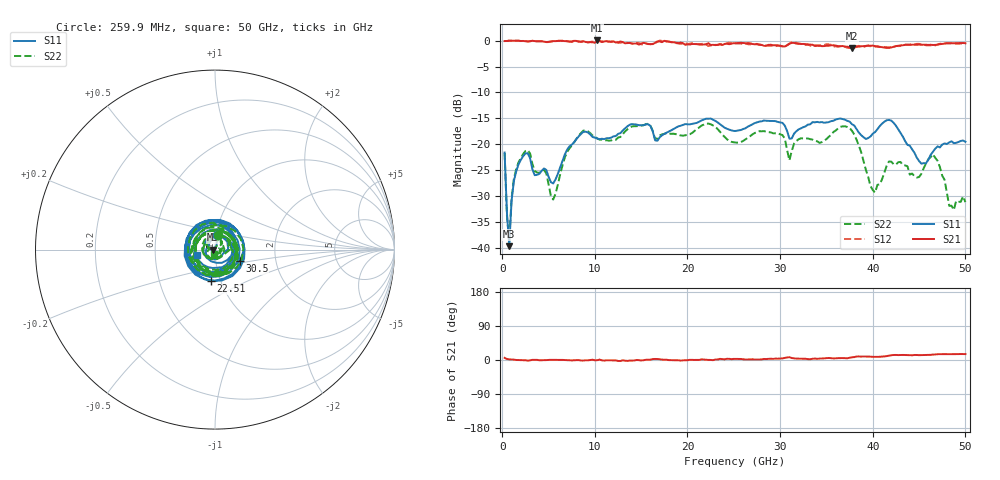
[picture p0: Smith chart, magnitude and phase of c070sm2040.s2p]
! 7/29/2020 12:24:18 PM
! D:\C070SM2040.S2P
! CHANNEL.1
! TR.MEASUREMENT
! CORRECTED.DATA
# GHZ S RI R 50.0
! FREQ.GHZ  S11RE  S11IM  S21RE  S21IM  S12RE  S12IM  S22RE  S22IM
!; PortSelection: Port_12
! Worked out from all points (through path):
!   200 points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, 259.9 MHz to 50 GHz, reference 50 ohm
!   highest |S21| = 0.03 dB at 10.26 GHz (marker M1); lowest = -1.5 dB at 37.75 GHz (marker M2)
!   lowest |S11| = -39.7 dB at 759.9 MHz (marker M3), VSWR 1.02, Z = 49 + j0.0382 ohm
!   |S11| at or under -10 dB: start of sweep to end of sweep
!   |S22| runs from -38.7 to -16.0 dB; largest |S21 - S12| = 0.057
!   S11 on the Smith chart (normalised r, x): 259.9 MHz: 1.01, +0.17; 22.51 GHz: 0.90, -0.33; 30.5 GHz: 1.31, -0.17; 50 GHz: 0.81, -0.05
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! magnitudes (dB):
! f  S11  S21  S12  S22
! 259.9 MHz  -21.6  -0.1  -0.1  -21.7
! 509.9 MHz  -33.2  -0.1  -0.1  -33.7
! 759.9 MHz  -39.7  0.0  0.0  -38.7
! 1.26 GHz  -27.1  0.0  0.0  -26.7
! 2.26 GHz  -22.3  -0.1  -0.1  -21.9
! 4.759 GHz  -25.0  -0.3  -0.3  -25.6
! 5.509 GHz  -27.6  -0.1  -0.1  -30.7
! 8.758 GHz  -17.6  -0.1  -0.2  -17.4
! 10.26 GHz  -18.9  0.0  -0.3  -18.9
! 17.01 GHz  -18.7  -0.2  0.0  -18.3
! 22.51 GHz  -15.0  -0.9  -0.9  -16.1
! 25.25 GHz  -17.4  -0.5  -0.5  -19.7
! 30.5 GHz  -16.4  -1.1  -1.1  -18.9
! 31 GHz  -18.9  -0.6  -0.6  -23.1
! 33.5 GHz  -15.7  -0.8  -1.0  -19.1
! 37.75 GHz  -16.1  -1.5  -1.2  -17.4
! 40.25 GHz  -17.6  -1.1  -1.1  -29.3
! 41.75 GHz  -15.3  -1.4  -1.3  -23.3
! 45.25 GHz  -23.7  -0.8  -0.8  -25.7
! 46.5 GHz  -21.4  -0.8  -0.8  -21.9
! 48.25 GHz  -19.7  -0.5  -0.5  -31.9
! 50 GHz  -19.5  -0.5  -0.5  -31.2
